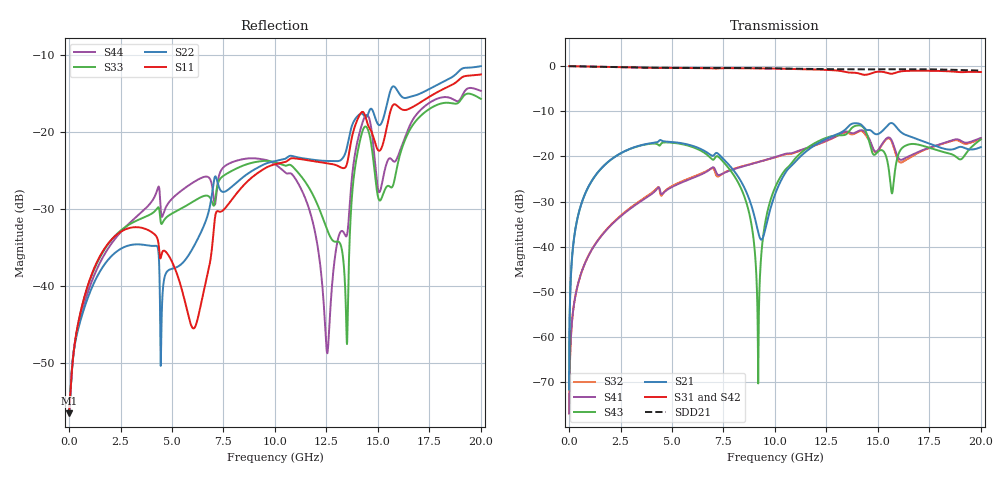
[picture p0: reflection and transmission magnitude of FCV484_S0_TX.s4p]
! Touchstone file from project M5P200_FCV484_DE158662_170512_85Ohm_120817
! Exported from HFSS 3D Layout Design 2017.2.0
! Port[1] = BGA.F21.SERDES_0_TX0_N
! Port[2] = BGA.F22.SERDES_0_TX0_P
! Port[3] = U1.410.SERDES_0_TX0_N
! Port[4] = U1.411.SERDES_0_TX0_P
# GHz S MA R 50
! freq  S11mag  S11ang  S12mag  S12ang  S13mag  S13ang  S14mag  S14ang
!  S21mag  S21ang  S22mag  S22ang  S23mag  S23ang  S24mag  S24ang
!  S31mag  S31ang  S32mag  S32ang  S33mag  S33ang  S34mag  S34ang
!  S41mag  S41ang  S42mag  S42ang  S43mag  S43ang  S44mag  S44ang
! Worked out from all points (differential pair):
!   4999 points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, 4.001 MHz to 20 GHz, reference 50 ohm
!   strongest paths, dB at 4.001 MHz, 5.001 GHz, 10 GHz, 15 GHz, 20 GHz:
!     S31: 0.0, -0.4, -0.5, -1.2, -1.3
!     S42: 0.0, -0.4, -0.6, -1.5, -1.4
!     S21: -71.5, -16.8, -28.4, -15.0, -17.9
!     S43: -71.5, -17.0, -26.9, -18.9, -16.2
!     S41: -76.8, -26.7, -20.1, -18.6, -15.9
!     S32: -76.8, -26.5, -20.2, -18.7, -16.1
!   taken as a pair (ports 1,2 in; 3,4 out), SDD21 dB: 0.0, -0.4, -0.5, -0.7, -1.0
!   lowest |S11| = -56.5 dB at 4.001 MHz (marker M1), VSWR 1.00, Z = 50.1 + j0.00996 ohm
!   |S11| at or under -10 dB: start of sweep to end of sweep
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0.0040008  0.00149 3.8  0.0002658 59.9  0.9985 -0.1  0.000144 -156.2
           0.0002658 59.9  0.001488 4.1  0.000144 -156.1  0.9985 -0.1
           0.9985 -0.1  0.000144 -156.1  0.00149 3.9  0.0002658 59.9
           0.000144 -156.2  0.9985 -0.1  0.0002658 59.9  0.001488 4.2
0.5281056  0.006478 -41.6  0.02652 77.9  0.9919 -10.6  0.004613 -107.5
           0.02652 77.9  0.005793 -33.2  0.004618 -107.4  0.9919 -10.7
           0.9919 -10.6  0.004618 -107.4  0.006473 -37.6  0.02653 77.5
           0.004613 -107.5  0.9919 -10.7  0.02653 77.5  0.006082 -28.5
2.704541  0.02325 -124.0  0.1145 37.8  0.9719 -52.8  0.02373 -139.2
          0.1145 37.8  0.01798 -131.2  0.02417 -139.0  0.972 -52.9
          0.9719 -52.8  0.02417 -139.0  0.02404 -102.8  0.1142 36.2
          0.02373 -139.2  0.972 -52.9  0.1142 36.2  0.0239 -89.7
7.609522  0.0324 -18.7  0.08829 -47.3  0.9493 -145.8  0.06707 121.3
          0.08829 -47.3  0.04133 -1.4  0.06761 121.0  0.948 -145.9
          0.9493 -145.8  0.06761 121.0  0.05324 -106.5  0.08138 -56.2
          0.06707 121.3  0.948 -145.9  0.08138 -56.2  0.06077 -116.0
9.185837  0.05457 -46.7  0.01455 -30.3  0.9448 -176.4  0.08686 93.5
          0.01455 -30.3  0.05906 -28.1  0.08695 91.7  0.9442 -176.8
          0.9448 -176.4  0.08695 91.7  0.06443 -126.3  0.0003081 172.8
          0.08686 93.5  0.9442 -176.8  0.0003081 172.8  0.06729 -141.9
11.4823  0.06609 -69.9  0.1122 47.8  0.9243 138.8  0.1229 48.9
         0.1122 47.8  0.06728 -51.8  0.1217 47.6  0.9237 138.1
         0.9243 138.8  0.1217 47.6  0.04732 -158.6  0.1206 43.3
         0.1229 48.9  0.9237 138.1  0.1206 43.3  0.03688 177.8
20  0.2372 -87.4  0.1271 -22.6  0.8594 -22.1  0.1603 -120.0
    0.1271 -22.6  0.2687 -83.0  0.1561 -122.4  0.8491 -22.7
    0.8594 -22.1  0.1561 -122.4  0.1647 -134.1  0.1547 135.0
    0.1603 -120.0  0.8491 -22.7  0.1547 135.0  0.1857 -144.5
